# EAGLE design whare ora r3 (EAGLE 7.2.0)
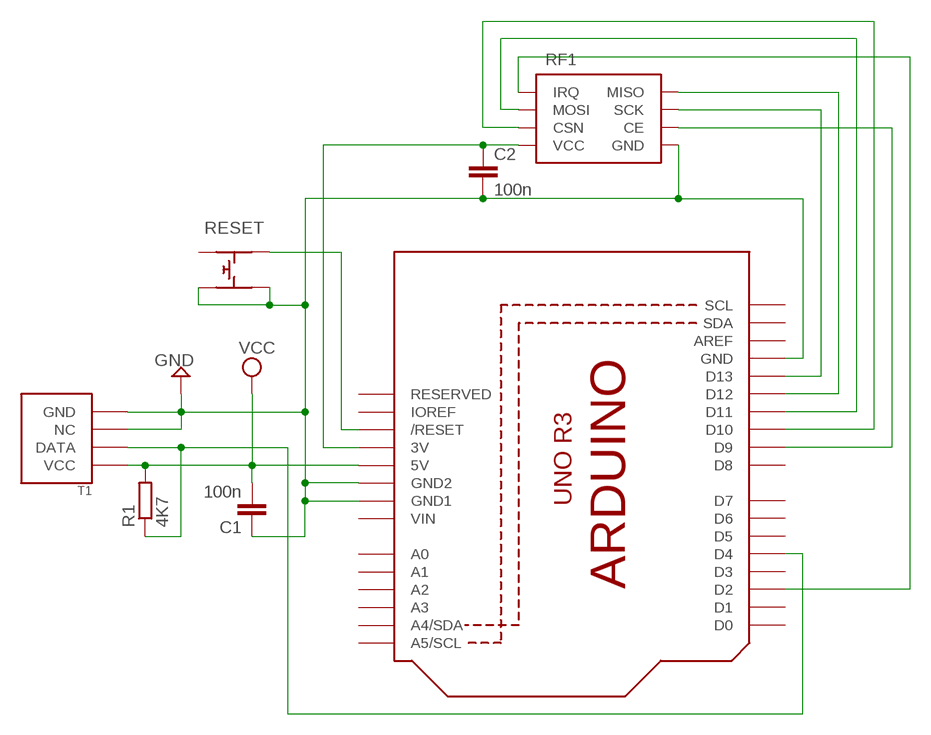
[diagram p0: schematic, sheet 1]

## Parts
C1  100n  C-EUC0805  [C0805]
C2  100n  C-EUC0805  [C0805]
R1  4K7  R-EU_M0805  [M0805]
RESET  SPST  [FSM-SMT]
RF1  NRF24L01+RF2  [RF2]
T1  DHT22  [DHT22]
U1  ARDUINOR3-DIMENSION  [ARDUINOR3]

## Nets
CE: RF1.P$3(CE) U1.D9
CS: RF1.P$4(CSN) U1.D10
GND: C1.1 C2.2 RESET.P$3 RESET.P$4 RF1.P$1(GND) T1.P$3(NC) T1.P$4(GND) U1.GND U1.GND1 U1.GND2
IRQ: RF1.P$8(IRQ) U1.D2
MISO: RF1.P$7(MISO) U1.D12
MOSI: RF1.P$6(MOSI) U1.D11
N$1: RESET.P$2 U1.RESET(/RESET)
N$2: R1.1 T1.P$2(DATA) U1.D4
SCK: RF1.P$5(SCK) U1.D13
VCC: C1.2 R1.2 T1.P$1(VCC) U1.5V
VDD: C2.1 RF1.P$2(VCC) U1.3V
Unconnected: RESET.P$1 U1.A0 U1.A1 U1.A2 U1.A3 U1.A4(A4/SDA) U1.A5(A5/SCL) U1.AREF U1.D0 U1.D1 U1.D3 U1.D5 U1.D6 U1.D7 U1.D8 U1.IOREF U1.RESERVED U1.SCL U1.SDA

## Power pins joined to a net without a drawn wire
VIN: U1.VIN

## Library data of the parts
C1 C2 = rcl:C-EU: CAPACITOR, European symbol
R1 = rcl:R-EU_: RESISTOR, European symbol
RESET = Callum:SPST
RF1 = Callum:NRF24L01+
T1 = Callum:DHT
U1 = adafruit:ARDUINOR3: This is a new object for the new Arduino R3 - with extra pins that you may want to use (such as IOref, and duplicated A4/A5

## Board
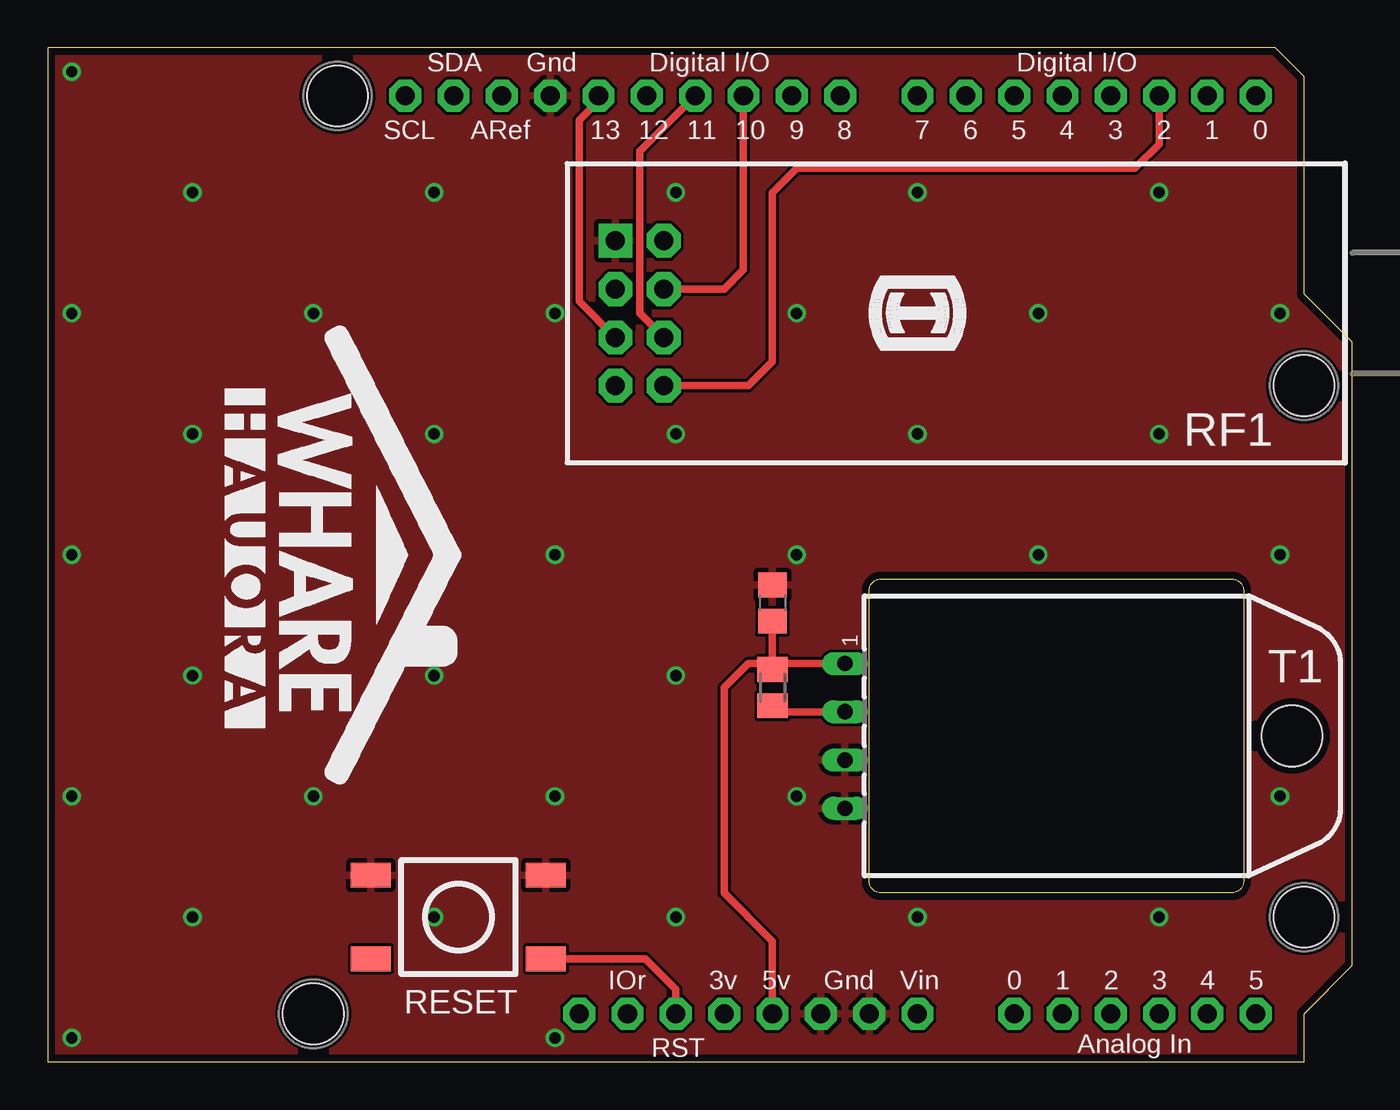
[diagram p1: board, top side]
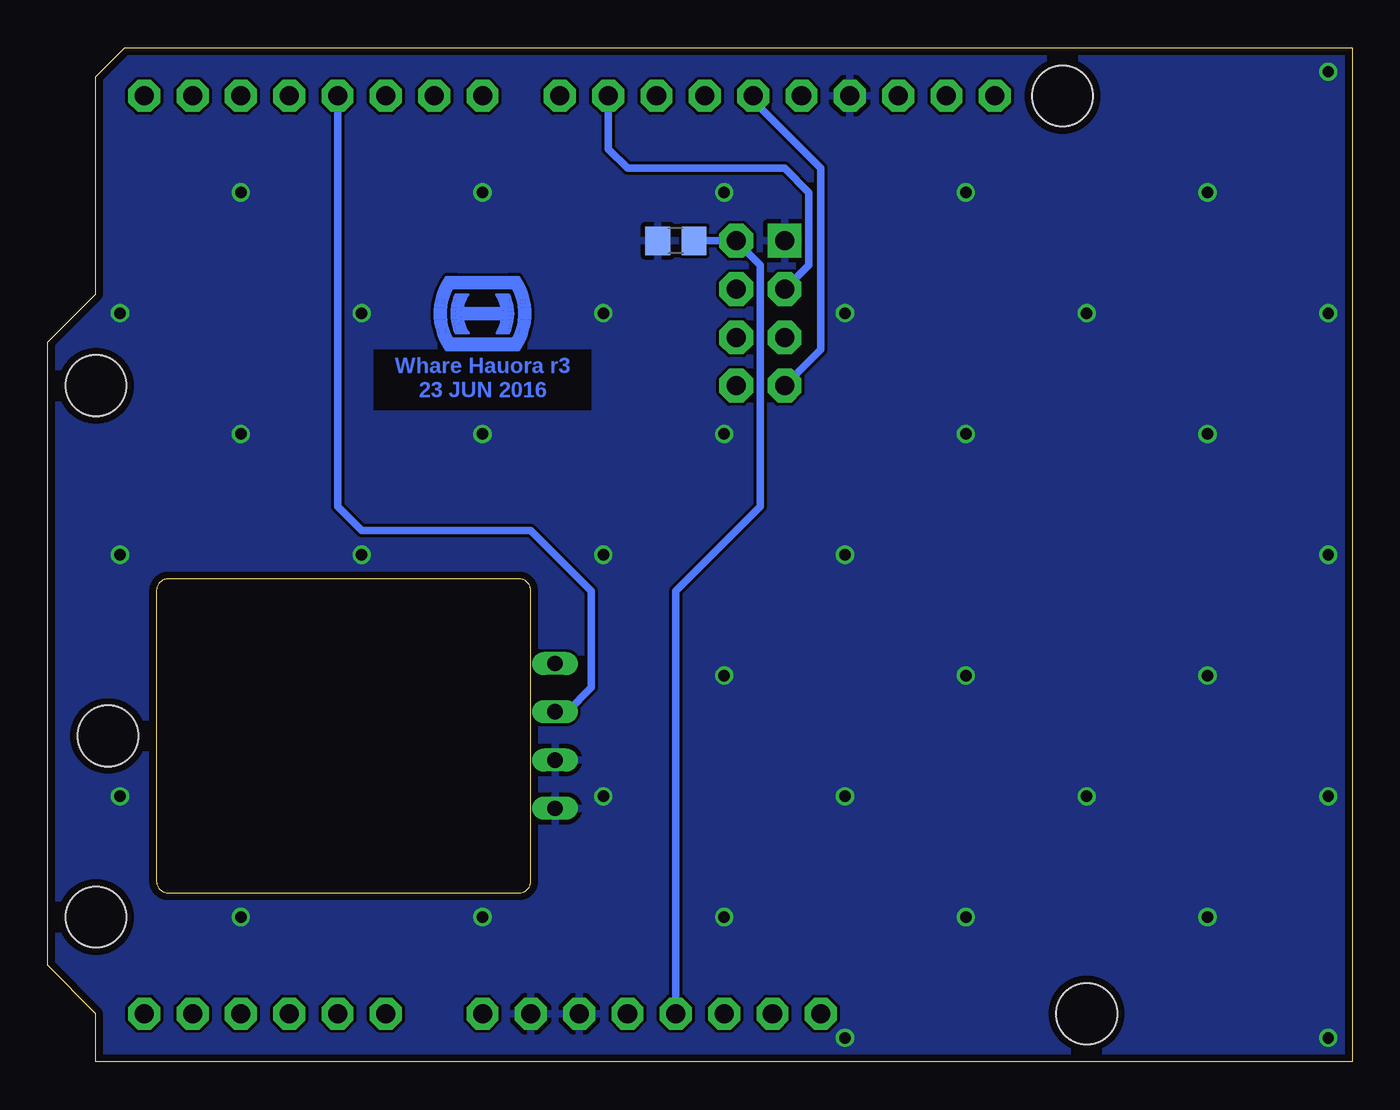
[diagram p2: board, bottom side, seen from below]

Size 68.58 x 53.34 mm. Coordinates in mm from the lower left corner, seen from the top.
Outline: 43.81,25.4 62.23,25.4 arc-90 62.87,24.77 62.87,9.53 arc-90 62.23,8.89 43.81,8.89 arc-90 43.18,9.53 43.18,24.77 arc-90 43.81,25.4
Copper layers (1*16): Top 0.0356mm / dielectric 1.5011mm / Bottom 0.0356mm
Design rules "OSHpark DRC *": minimum track width 6mil, minimum drill 13mil, track to track 6mil, track to pad 6mil, pad to pad 6mil, via to via 6mil, smd to smd 6mil, copper to edge 15mil, drill to drill 6mil, minimum pad ring 7mil, minimum via ring 7mil, stop-mask expansion 3mil, vias tented up to drill 30mil, thermal gap 10mil
Holes 3.2 mm at 66.04,35.56 66.04,7.62 13.97,2.54 15.24,50.8
bRestrict: area 40,34.3 to 51.4,37.5

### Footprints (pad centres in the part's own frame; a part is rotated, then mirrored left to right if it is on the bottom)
C0805 = smd 1.3 x 1.5: 1 -0.95,0; 2 0.95,0
M0805 = smd 1.3 x 1.6: 1 -0.95,0; 2 0.95,0
FSM-SMT = smd 1.3 x 2.1: P$1 -2.2,4.6; P$2 -2.2,-4.6; P$3 2.2,4.6; P$4 2.2,-4.6
RF2 = drill 1 pad 1.778 square: P$1 0,0 | drill 1 pad 1.778 octagon: P$2 -2.54,0; P$3 0,2.54; P$4 -2.54,2.54; P$5 0,5.08; P$6 -2.54,5.08; P$7 0,7.62; P$8 -2.54,7.62
DHT22 = drill 0.8 long: P$1 0,0; P$2 2.54,0; P$3 5.08,0; P$4 7.62,0 | hole 3.2: 3.81,23.495
ARDUINOR3 = drill 1 pad 1.676 octagon: 3V 35.56,2.54; 5V 38.1,2.54; A0 50.8,2.54; A1 53.34,2.54; A2 55.88,2.54; A3 58.42,2.54; A4 60.96,2.54; A5 63.5,2.54; AREF 23.876,50.8; D0 63.5,50.8; D1 60.96,50.8; D2 58.42,50.8; D3 55.88,50.8; D4 53.34,50.8; D5 50.8,50.8; D6 48.26,50.8; D7 45.72,50.8; D8 41.656,50.8; D9 39.116,50.8; D10 36.576,50.8; D11 34.036,50.8; D12 31.496,50.8; D13 28.956,50.8; GND 26.416,50.8; GND1 43.18,2.54; GND2 40.64,2.54; IOREF 30.48,2.54; RESERVED 27.94,2.54; RESET 33.02,2.54; SCL 18.796,50.8; SDA 21.336,50.8; VIN 45.72,2.54

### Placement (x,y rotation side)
C1  38.1,24.13 270 top
C2  35.56,43.18 180 bottom
R1  38.1,19.68 90 top
RESET  21.59,7.62 90 top
RF1  29.84,43.18 180 top
T1  41.91,20.95 270 top
U1  0,0 0 top
U$1  [MY-LOGO-COPPER]  45.72,39.37 0 bottom
U$2  [MY-LOGO-SMALL]  45.72,39.37 180 top
U$3  [WHAREHAUORA]  9.53,38.1 270 top

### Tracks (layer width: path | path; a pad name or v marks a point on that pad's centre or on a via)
CE
  Bottom 0.406: RF1.P$3 28.57,41.91 28.57,45.72 29.84,46.99 38.1,46.99 39.12,48.01 U1.D9
CS
  Top 0.406: U1.D10 36.58,41.66 35.56,40.64 RF1.P$4
GND  (via drill 0.6)
  other vias: 1.27,1.27 1.27,52.07 1.27,39.37 1.27,13.97 1.27,26.67 64.77,13.97 64.77,26.67 7.62,45.72 7.62,7.62 13.97,13.97 13.97,39.37 20.32,45.72 20.32,33.02 20.32,20.32 20.32,7.62 26.67,39.37 26.67,26.67 26.67,13.97 39.37,13.97 33.02,33.02 45.72,33.02 58.42,33.02 52.07,39.37 45.72,45.72 64.77,39.37 39.37,39.37 33.02,7.62 45.72,7.62 58.42,7.62 52.07,26.67 33.02,20.32 58.42,45.72 39.37,26.67 7.62,33.02 7.62,20.32 33.02,45.72 26.67,1.27
  pour Bottom: 0,0 66.04,0 66.04,2.54 68.58,5.08 68.58,13.34 68.58,29.84 68.58,38.1 66.04,40.64 66.04,52.07 64.77,53.34 0,53.34
  pour Top: 0,53.34 64.77,53.34 66.04,52.07 66.04,40.64 68.58,38.1 68.58,29.84 68.58,13.34 68.58,5.08 66.04,2.54 66.04,0 0,0
IRQ
  Top 0.406: U1.D2 58.42,48.26 57.15,46.99 39.37,46.99 38.1,45.72 38.1,36.83 36.83,35.56 RF1.P$8
MISO
  Bottom 0.406: RF1.P$7 27.94,37.47 27.94,46.99 31.5,50.55 U1.D12
MOSI
  Top 0.406: RF1.P$6 31.11,39.37 31.11,47.88 U1.D11
N$1
  Top 0.406: U1.RESET 33.02,3.81 31.41,5.42 RESET.P$2
N$2
  Top 0.406: T1.P$2 38.42,18.41 R1.1
  Bottom 0.406: U1.D4 53.34,29.21 52.07,27.94 43.18,27.94 40.01,24.77 40.01,19.68 41.27,18.41 T1.P$2
SCK
  Top 0.406: U1.D13 28.96,50.55 27.94,49.53 27.94,40.01 RF1.P$5
VCC
  Top 0.406: U1.5V 38.1,6.35 35.56,8.89 35.56,19.68 36.83,20.95 38.1,20.95 | T1.P$1 38.1,20.95 | 38.1,20.95 R1.2 C1.2
VDD
  Bottom 0.406: U1.3V 35.56,24.77 31.11,29.21 31.11,41.91 RF1.P$2 C2.1

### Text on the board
Bottom: Whare Hauora r3 | 23 JUN 2016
